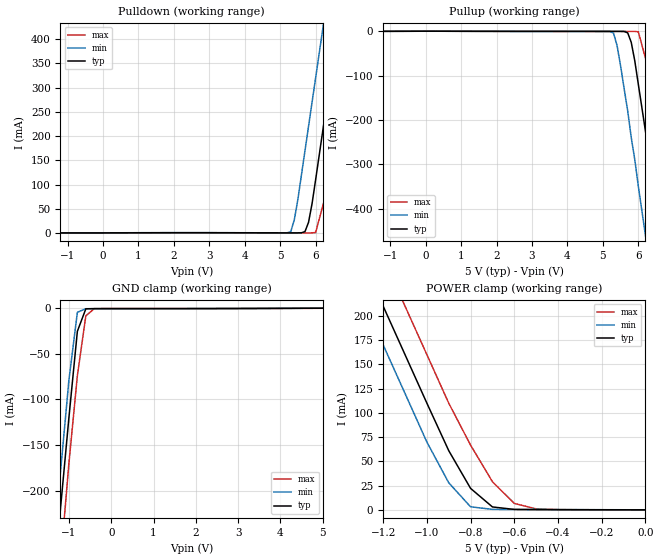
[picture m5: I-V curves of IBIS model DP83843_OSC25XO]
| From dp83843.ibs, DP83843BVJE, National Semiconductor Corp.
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|   Model OSC25XO
[Model]   DP83843_OSC25XO
Model_type   I/O
Polarity   Inverting
Enable   Active-High
Vinl =   0.80V
Vinh =   2.00V
Vmeas =   1.50V
Cref =  10.00pF
Rref =  50.00
C_comp   5.83pF   5.83pF   5.83pF
[Temperature Range]   50.00   -15.00   0.15k
[Voltage Range]   5.00V   4.50V   5.50V
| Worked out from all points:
|   slope of the pulldown table from 0 to 0.75 V, typ, clamps not added: 4.69 kohm
|   slope of the pullup table from 0 to 0.75 V, typ, clamps not added: 7.3 kohm
|   GND clamp passes 1 mA (typ) near -0.60 V on its own axis
|   POWER clamp passes 1 mA (typ) near -0.62 V on its own axis
[Pulldown]
| voltage   I(typ)   I(min)   I(max)
-5V       470uA      550uA      410uA
5.3V      460uA      3.24mA     340uA
5.4V      460uA      27.98mA    340uA
5.5V      470uA      69.88mA    340uA
5.7V      3.13mA     170mA      340uA
5.8V      22.19mA    220mA      350uA
5.9V      61.07mA    270mA      420uA
6V        110mA      320mA      1.19mA
6.4V      310mA      520mA      110mA
6.8V      520mA      730mA      310mA
7.2V      740mA      940mA      520mA
10V       2.26A      2.41A      2.03A
[Pullup]
| voltage   I(typ)   I(min)   I(max)
-5V       -670uA     -770uA     -600uA
5.2V      -420uA     -610uA     -360uA
5.3V      -420uA     -4.37mA    -360uA
5.4V      -430uA     -32.57mA   -360uA
5.7V      -3.78mA    -180mA     -370uA
5.8V      -25.16mA   -240mA     -370uA
5.9V      -67.12mA   -290mA     -450uA
6V        -120mA     -350mA     -1.41mA
6.4V      -330mA     -570mA     -120mA
6.8V      -560mA     -800mA     -340mA
7.2V      -790mA     -1.03A     -560mA
10V       -2.42A     -2.63A     -2.18A
[GND_clamp]
| voltage   I(typ)   I(min)   I(max)
-5V       -2.42A     -2.35A     -2.47A
-1.4V     -340mA     -290mA     -390mA
-1.2V     -220mA     -180mA     -280mA
-1V       -120mA     -78.9mA    -170mA
-800mV    -25.3mA    -4.48mA    -73.93mA
-600mV    -670uA     -560uA     -8.38mA
-400mV    -470uA     -560uA     -500uA
5V        42.03pA    150uA      -78.61uA
[POWER_clamp]
| voltage   I(typ)   I(min)   I(max)
-5V       2.26A      2.15A      2.31A
-1.3V     260mA      220mA      310mA
-1.2V     210mA      170mA      260mA
-1.1V     160mA      120mA      210mA
-1V       110mA      69.9mA     160mA
-900mV    61.05mA    27.95mA    110mA
-800mV    22.14mA    3.16mA     66.73mA
-700mV    3.03mA     540uA      29.01mA
-600mV    470uA      420uA      6.69mA
-500mV    280uA      360uA      1.05mA
0V        45.56uA    58.19uA    31.74uA
[Ramp]
| variable   typ   min   max
dV/dt_r   11.19m/0.24n   12.85m/0.18n   9.93m/0.36n
dV/dt_f   12.38m/0.27n   16.19m/0.22n   9.35m/0.33n
R_load = 50.00
| End [Model] OSC25XO
